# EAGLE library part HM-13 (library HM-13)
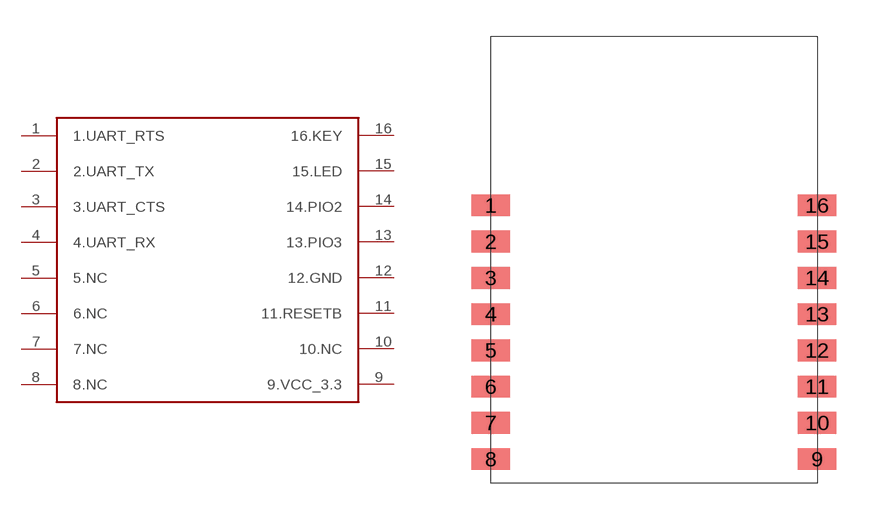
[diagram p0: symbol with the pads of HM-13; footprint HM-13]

Designator prefix -

## HM-13  [HM-13]
1  1.UART_RTS
2  2.UART_TX
3  3.UART_CTS
4  4.UART_RX
5  5.NC
6  6.NC
7  7.NC
8  8.NC
9  9.VCC_3.3
10  10.NC
11  11.RESETB
12  12.GND
13  13.PIO3
14  14.PIO2
15  15.LED
16  16.KEY

## Footprint HM-13 (pad centres in mm)
smd 1.6 x 0.9: 1 0,11.5; 2 0,10; 3 0,8.5; 4 0,7; 5 0,5.5; 6 0,4; 7 0,2.5; 8 0,1; 9 13.5,1; 10 13.5,2.5; 11 13.5,4; 12 13.5,5.5; 13 13.5,7; 14 13.5,8.5; 15 13.5,10; 16 13.5,11.5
